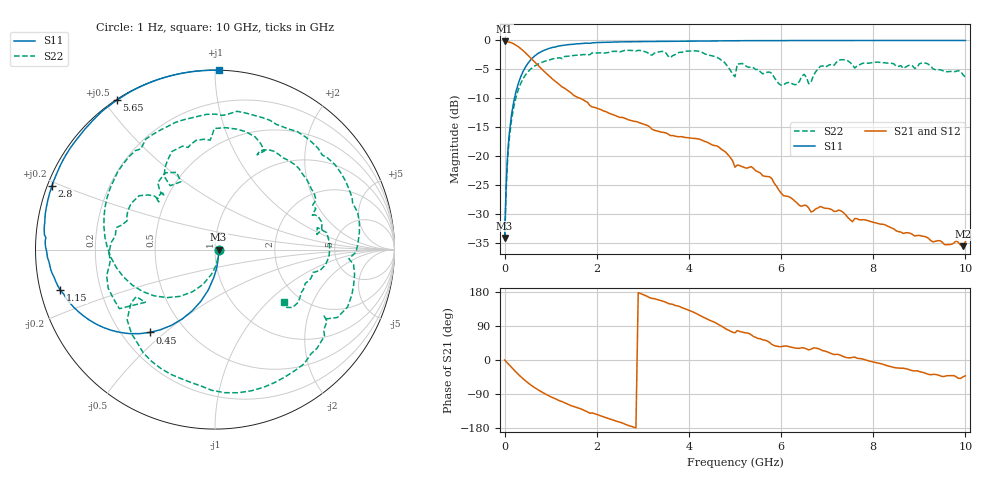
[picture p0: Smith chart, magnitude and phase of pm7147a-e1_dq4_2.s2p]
# GHz S DB R 50
! S-Parameters data
! Freq  dbS11  angS11  dbS21  angS21  dbS12  angS12  dbS22  angS22
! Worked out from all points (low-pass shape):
!   279 points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, 1 Hz to 10 GHz, reference 50 ohm
!   highest |S21| = -0.17 dB at 158.5 Hz (marker M1); lowest = -35.5 dB at 9.95 GHz (marker M2)
!   |S21| within 3 dB of the highest: start of sweep to 583.2 MHz
!   lowest |S11| = -34.1 dB at 3.2 Hz (marker M3), VSWR 1.04, Z = 52 - j3.89e-07 ohm
!   |S11| at or under -10 dB: start of sweep to 213.9 MHz
!   |S22| runs from -34.1 to -1.7 dB; largest |S21 - S12| = 0
!   S11 on the Smith chart (normalised r, x): 1 Hz: 1.04, -0.00; 450 MHz: 0.32, -0.45; 1.15 GHz: 0.06, -0.13; 2.8 GHz: 0.01, +0.19; 5.65 GHz: 0.00, +0.54; 10 GHz: 0.00, +1.03
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1e-09  -34.08 -0.0  -0.17 -0.0  -0.17 -0.0  -34.08 -0.0
3.2e-09  -34.08 -0.0  -0.17 -0.0  -0.17 -0.0  -34.08 -0.0
1.585e-07  -34.08 -0.0  -0.17 -0.0  -0.17 -0.0  -34.08 -0.0
0.06309573  -20.05 -84.4  -0.22 -8.3  -0.22 -8.3  -20.86 -87.6
0.15  -12.83 -99.5  -0.42 -19.7  -0.42 -19.7  -13.71 -109.1
0.45  -4.62 -128.2  -2.12 -54.7  -2.12 -54.7  -5.98 -157.0
0.75  -2.13 -148.0  -4.52 -80.5  -4.52 -80.5  -3.99 168.4
1.15  -1.01 -165.2  -7.36 -105.2  -7.36 -105.2  -3.03 132.9
1.7  -0.51 179.3  -10.22 -131.6  -10.22 -131.6  -2.44 93.4
2.3  -0.29 167.1  -12.65 -156.2  -12.65 -156.2  -1.92 55.2
2.8  -0.21 158.6  -13.94 -177.3  -13.94 -177.3  -1.76 20.8
3.35  -0.16 150.5  -15.69 158.2  -15.69 158.2  -1.97 -14.3
4.2  -0.13 139.4  -16.98 120.1  -16.98 120.1  -1.85 -80.8
4.65  -0.09 134.2  -18.39 92.8  -18.39 92.8  -3.09 -124.8
5.05  -0.05 129.7  -21.48 77.7  -21.48 77.7  -4.06 -148.3
5.65  -0.03 123.2  -23.44 52.4  -23.44 52.4  -5.63 160.2
6.7  -0.01 113.1  -29.44 31.9  -29.44 31.9  -6.09 124.7
7.3  -0.01 107.9  -29.40 11.8  -29.40 11.8  -3.33 85.1
8.35  -0.00 99.6  -32.17 -16.6  -32.17 -16.6  -3.96 32.2
9.15  -0.00 94.0  -33.90 -35.7  -33.90 -35.7  -3.93 -3.5
9.95  -0.00 88.9  -35.49 -44.3  -35.49 -44.3  -5.94 -39.6
10  -0.00 88.6  -34.67 -41.8  -34.67 -41.8  -6.36 -37.1
